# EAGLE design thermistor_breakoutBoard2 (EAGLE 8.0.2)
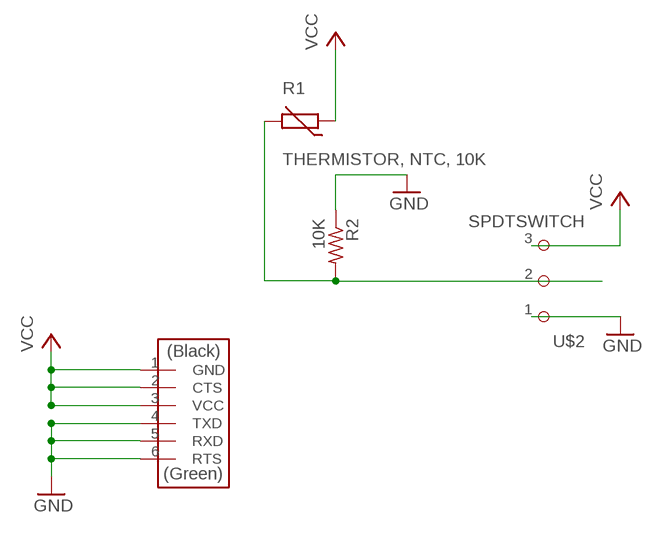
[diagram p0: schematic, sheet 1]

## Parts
R1  THERMISTOR, NTC, 10K  THERMISTOR-2,5  [RS-2,5]
R2  10K  RES-US1206FAB  [R1206FAB]
U$1  FTDI-SMD-HEADER  [1X06SMD]
U$2  SPDTSWITCH  [SPDTSWITCH]

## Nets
GND: R2.1 U$1.4(TXD) U$1.5(RXD) U$1.6(RTS) U$2.1
INPUT: R1.2 R2.2 U$2.2
VCC: R1.1 U$1.1(GND) U$1.2(CTS) U$1.3(VCC) U$2.3

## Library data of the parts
R1 = varistor:THERMISTOR: THERMISTOR
R2 = fab:RES-US: Resistor (US Symbol)
U$1 = fab:FTDI-SMD-HEADER
U$2 = fab:SPDTSWITCH

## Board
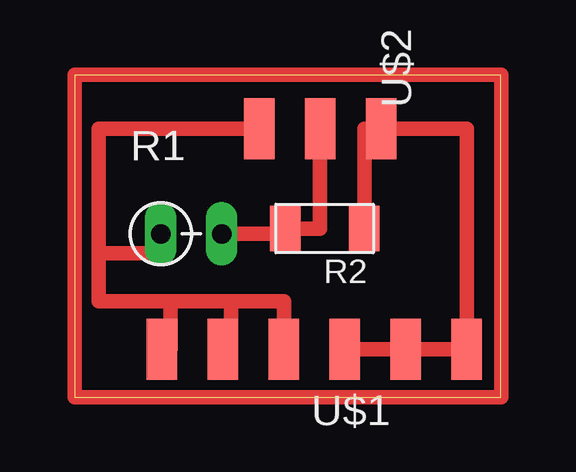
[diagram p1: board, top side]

Size 17.78 x 13.42 mm. Coordinates in mm from the lower left corner, seen from the top.
Outline: 0,0 17.78,0 17.78,13.42 0,13.42 0,0
Copper layers (1*16): Top 0.035mm / dielectric 1.5mm / Bottom 0.035mm
Design rules "default": minimum track width 10mil, minimum drill 24mil, track to track 8mil, track to pad 8mil, pad to pad 8mil, via to via 8mil, smd to smd 8mil, copper to edge 40mil, drill to drill 8mil, minimum pad ring 10mil, minimum via ring 8mil, stop-mask expansion 4mil, vias tented up to drill 0mil, thermal gap 10mil

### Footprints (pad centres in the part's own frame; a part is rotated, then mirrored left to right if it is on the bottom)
RS-2,5 = drill 0.813 long: 1 -1.27,0; 2 1.27,0
R1206FAB = smd 1.27 x 1.905: 1 -1.651,0; 2 1.651,0
1X06SMD = smd 2.54 x 1.27: 1 0,6.35; 2 0,3.81; 3 0,1.27; 4 0,-1.27; 5 0,-3.81; 6 0,-6.35
SPDTSWITCH = smd 2.54 x 1.27: 1 0.38,2.54; 2 0.38,0; 3 0.38,-2.54

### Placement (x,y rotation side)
R1  4.87,6.81 0 top
R2  10.43,7.03 180 top
U$1  10,2 90 top
U$2  10.24,11.57 270 top

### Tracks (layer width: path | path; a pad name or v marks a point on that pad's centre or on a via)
GND
  Top 0.61: 12.27,7.03 R2.1 12.08,11.19 U$2.1 16.35,11.19 U$1.6 U$1.5 U$1.4
INPUT
  Top 0.61: 9,7.03 R2.2 | R1.2 8.78,6.81 R2.2 | R2.2 10.24,7.03 U$2.2
N$2
  Top 0.61: 0,0 17.8,0 17.8,13.45 0,13.45 0,0.03
VCC
  Top 0.61: U$2.3 1,11.19 1,6 | 1,6 1,4 4,4 | 1,6 3.6,6 R1.1 | 4,4 6.53,4 | 6.53,4 8.73,4 U$1.3 | U$1.2 6.53,2 6.53,4 | U$1.1 4,2 4,4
